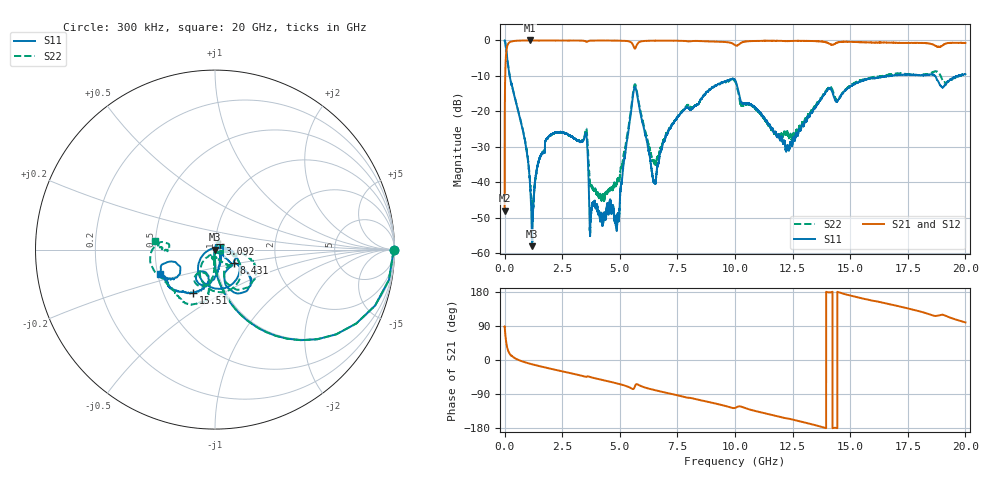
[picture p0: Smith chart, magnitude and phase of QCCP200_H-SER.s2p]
!{QCCP200}
!Johanson Technology Inc.
!www.johansontechnology.com
!Test Board Conditions:
!Substrate Type  RO4350B
!Substrate Thickness  20 mil
!Substrate Dk  3.66
!TL Type: GCPW
!TL Trace Width  36 mil
!TL Gap  12 mil
!Electrode orientation  Horizontal
!DUT TOPOLOGY	SERIES
!Mounting Pad LxW  26x36 mil
! Created Sat Jan  9 18:33:26 2021
# hz S ma R 50
! 2 Port Network Data from SP1.SP block
! freq  magS11  angS11  magS21  angS21  magS12  angS12  magS22  angS22
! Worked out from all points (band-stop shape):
!   20001 points, 300 kHz to 20 GHz, reference 50 ohm
!   highest |S21| = 0.00 dB at 1.114 GHz (marker M1); lowest = -48.1 dB at 300 kHz (marker M2)
!   |S21| within 3 dB of the highest: 76.79 MHz to end of sweep
!   lowest |S11| = -58.1 dB at 1.193 GHz (marker M3), VSWR 1.00, Z = 49.9 + j0.00551 ohm
!   |S11| at or under -10 dB: 221 MHz to 16.7 GHz (16.48 GHz wide, 195 % of centre); 16.77434 GHz to 16.79774 GHz (23.39 MHz wide, 0.139 % of centre); 18.69 GHz to 19.69 GHz (999.7 MHz wide, 5.21 % of centre)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
!   |S22| runs from -50.7 to 0.0 dB; largest |S21 - S12| = 0.017
!   S11 on the Smith chart (normalised r, x): 300 kHz: open; 3.092 GHz: 1.05, +0.07; 8.431 GHz: 1.23, -0.18; 15.51 GHz: 0.70, -0.37; 20 GHz: 0.52, -0.16
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300000  0.9949 -0.2  0.00395 88.7  0.003895 89.1  0.9957 -0.2
1.493e8  0.4478 -64.6  0.8899 25.3  0.8904 25.1  0.451 -64.3
9.013e8  0.03535 -96.6  0.9978 -6.3  0.9978 -6.3  0.03679 -92.9
1.1143e9  0.008027 -110.4  0.9995 -10.0  0.9986 -10.0  0.009296 -83.2
1.1933e9  0.001245 177.5  0.9981 -11.3  0.9986 -11.2  0.003613 -36.4
1.8503e9  0.04128 65.2  0.9976 -21.0  0.9972 -21.0  0.04093 73.1
3.0923e9  0.04021 50.5  0.9955 -37.9  0.9959 -37.9  0.04019 54.4
3.3343e9  0.03739 46.2  0.995 -41.3  0.9943 -41.3  0.03842 46.4
3.5363e9  0.04916 4.3  0.9633 -44.6  0.9638 -44.6  0.05676 8.6
3.7513e9  0.003704 53.6  0.9942 -45.6  0.9946 -45.6  0.008974 -17.1
4.2143e9  0.003473 135.3  0.9969 -52.3  0.9973 -52.3  0.005781 -47.0
4.8993e9  0.003272 77.2  0.9937 -62.1  0.9942 -62.1  0.01068 -49.9
5.6533e9  0.2211 -74.6  0.7653 -70.1  0.7659 -70.1  0.2414 -73.1
6.4603e9  0.01046 128.1  0.9918 -78.6  0.9921 -78.6  0.02026 -91.3
6.6673e9  0.0181 40.6  0.9934 -81.6  0.9931 -81.6  0.02249 -37.4
8.4313e9  0.1298 -34.2  0.9826 -105.2  0.9811 -105.1  0.1309 -4.6
1.00003e10  0.2768 -62.0  0.8596 -126.6  0.8592 -126.5  0.2639 -57.1
1.22713e10  0.03238 -39.2  0.9777 -154.2  0.9778 -154.2  0.05204 -109.0
1.33343e10  0.09587 -75.1  0.9801 -169.7  0.9836 -169.6  0.1025 -90.8
1.55123e10  0.2699 -116.8  0.943 162.8  0.9502 162.7  0.2771 -100.0
1.66673e10  0.3122 -133.2  0.931 147.8  0.9252 147.6  0.3302 -112.4
2e10  0.3335 -155.6  0.9195 99.2  0.9103 99.1  0.3404 171.9
